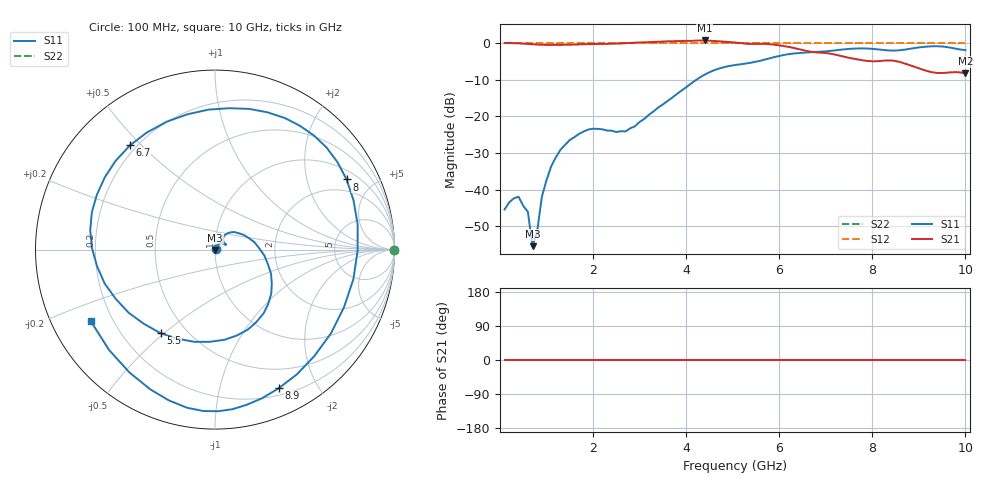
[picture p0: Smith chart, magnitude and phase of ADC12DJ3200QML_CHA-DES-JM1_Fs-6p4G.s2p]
!	Texas	"Instruments,"	Inc.
!	ADC12DJ3200	-	CH	A	S-Parameters	(DES	"Mode,"	Fs	=	6.4	"GSPS,"	25	degC	"case,"	15	degC	juntion)
!	Port	1	represents	the	100-ohm	differenal	"input,"	Port	2	the	digital	output
!	freq	dbS11	angS11	dbS21	angS21	dbS12	angS12	dbS22	angS22
#	HZ	S	DB	R	100
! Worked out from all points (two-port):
!   100 points, 100 MHz to 10 GHz, reference 100 ohm
!   highest |S21| = 0.68 dB at 4.4 GHz (marker M1); lowest = -8.3 dB at 10 GHz (marker M2)
!   |S21| within 3 dB of the highest: start of sweep to 6.645 GHz
!   lowest |S11| = -55.4 dB at 700 MHz (marker M3), VSWR 1.00, Z = 100 - j0.338 ohm
!   |S11| at or under -10 dB: start of sweep to 4.226 GHz
!   |S22| runs from 0.0 to 0.0 dB; largest |S21 - S12| = 0.62
!   S11 on the Smith chart (normalised r, x): 100 MHz: 1.01, +0.00; 5.5 GHz: 0.36, -0.49; 6.7 GHz: 0.17, +0.46; 8 GHz: 1.38, +3.49; 8.9 GHz: 0.27, -1.52; 10 GHz: 0.12, -0.26
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1e8  -45.42 10.5  0.00 0.0  0.00 0.0  0.00 0.0
4e8  -41.94 -35.7  -0.10 0.0  0.00 0.0  0.00 0.0
6e8  -46.07 -54.1  -0.25 0.0  0.00 0.0  0.00 0.0
7e8  -55.43 -89.2  -0.35 0.0  0.00 0.0  0.00 0.0
8e8  -51.37 26.7  -0.42 0.0  0.00 0.0  0.00 0.0
9e8  -41.96 75.7  -0.49 0.0  0.00 0.0  0.00 0.0
1.1e9  -33.67 69.2  -0.54 0.0  0.00 0.0  0.00 0.0
1.8e9  -24.15 33.6  -0.35 0.0  0.00 0.0  0.00 0.0
2.7e9  -24.14 41.3  -0.05 0.0  0.00 0.0  0.00 0.0
3.4e9  -17.60 47.1  0.32 0.0  0.00 0.0  0.00 0.0
4.4e9  -8.63 -31.2  0.68 0.0  0.00 0.0  0.00 0.0
5.1e9  -5.93 -84.0  0.06 0.0  0.00 0.0  0.00 0.0
5.5e9  -5.10 -123.1  -0.27 0.0  0.00 0.0  0.00 0.0
6.1e9  -3.28 179.2  -0.87 0.0  0.00 0.0  0.00 0.0
6.7e9  -2.50 129.2  -2.45 0.0  0.00 0.0  0.00 0.0
7.3e9  -1.86 76.3  -3.47 0.0  0.00 0.0  0.00 0.0
8e9  -1.61 28.1  -5.00 0.0  0.00 0.0  0.00 0.0
8.4e9  -2.07 -12.1  -4.77 0.0  0.00 0.0  0.00 0.0
8.9e9  -1.41 -65.3  -6.47 0.0  0.00 0.0  0.00 0.0
9.5e9  -0.96 -99.9  -8.19 0.0  0.00 0.0  0.00 0.0
9.8e9  -1.57 -124.9  -7.97 0.0  0.00 0.0  0.00 0.0
1e10  -1.95 -150.1  -8.32 0.0  0.00 0.0  0.00 0.0
